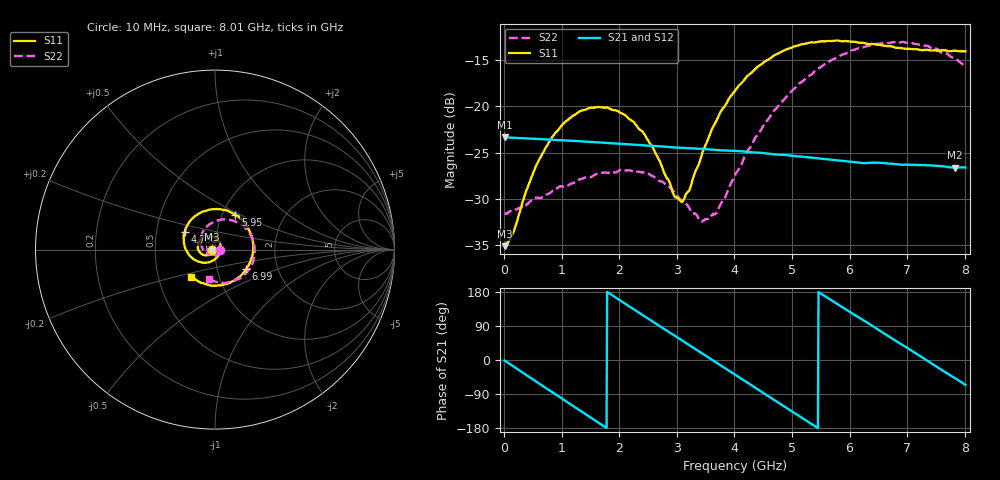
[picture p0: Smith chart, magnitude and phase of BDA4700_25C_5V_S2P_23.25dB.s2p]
!Agilent Technologies,E5071B,MY42404982,A.09.10
!Date: Mon Oct 20 13:38:07 2025
!Data & Calibration Information:
!Freq	S11:SOLT2(ON)	S21:SOLT2(ON)	S12:SOLT2(ON)	S22:SOLT2(ON)
# Hz S RI R 50
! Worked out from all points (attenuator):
!   801 points, 10 MHz to 8.01 GHz, reference 50 ohm
!   highest |S21| = -23.33 dB at 10 MHz (marker M1); lowest = -26.6 dB at 7.83 GHz (marker M2)
!   lowest |S11| = -35.2 dB at 10 MHz (marker M3), VSWR 1.04, Z = 48.3 - j0.102 ohm
!   |S11| at or under -10 dB: start of sweep to end of sweep
!   |S22| runs from -32.5 to -13.0 dB; largest |S21 - S12| = 0.00049
!   S11 on the Smith chart (normalised r, x): 10 MHz: 0.97, -0.00; 4.79 GHz: 0.70, +0.14; 5.95 GHz: 1.15, +0.47; 6.99 GHz: 1.38, -0.32; 8.01 GHz: 0.74, -0.23
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1e7  -0.0174 -0.00105  0.0682 -0.00146  0.0682 -0.00154  0.0262 -0.000834
1.6e8  -0.0183 -0.00974  0.0648 -0.0193  0.0648 -0.0193  0.0263 -0.0075
4.3e8  -0.0282 -0.0251  0.0482 -0.0466  0.0482 -0.0466  0.0196 -0.0227
7.3e8  -0.0508 -0.0322  0.0179 -0.0637  0.0179 -0.0638  0.00382 -0.033
1.35e9  -0.095 0.00575  -0.0469 -0.0445  -0.0469 -0.0445  -0.0364 -0.0177
2.09e9  -0.05 0.0751  -0.0541 0.0313  -0.0541 0.0314  -0.0289 0.0346
2.42e9  -0.0071 0.0717  -0.0282 0.0547  -0.0282 0.0547  -0.00428 0.0437
2.68e9  0.0198 0.0481  -0.00183 0.0608  -0.0019 0.0608  0.0136 0.0373
2.96e9  0.0311 0.00969  0.0259 0.054  0.026 0.0539  0.0261 0.022
3.1e9  0.0284 -0.0112  0.0379 0.0461  0.0378 0.0461  0.0284 0.0107
3.41e9  0.00121 -0.0515  0.0552 0.0204  0.0553 0.0204  0.0204 -0.0124
3.54e9  -0.017 -0.0638  0.0581 0.00763  0.0581 0.00757  0.0127 -0.0211
3.7e9  -0.0457 -0.0718  0.0575 -0.00815  0.0574 -0.00829  -0.00111 -0.0268
4.01e9  -0.1049 -0.0612  0.0449 -0.0357  0.0449 -0.0357  -0.033 -0.0263
4.79e9  -0.169 0.0988  -0.0233 -0.0495  -0.0231 -0.0497  -0.0793 0.0662
5.35e9  -0.0669 0.2117  -0.0519 -0.00913  -0.0519 -0.0093  -0.0155 0.1491
5.95e9  0.1139 0.1951  -0.0337 0.0376  -0.0338 0.0374  0.1207 0.1526
6.68e9  0.2118 -0.0137  0.0229 0.0433  0.0229 0.0434  0.2207 -0.00147
6.99e9  0.173 -0.1103  0.0406 0.0262  0.0407 0.0261  0.2041 -0.0851
7.43e9  0.0516 -0.1943  0.0471 -0.00802  0.0471 -0.0082  0.1177 -0.1691
7.83e9  -0.0811 -0.1835  0.0312 -0.0346  0.0311 -0.0348  0.0109 -0.1812
8.01e9  -0.1311 -0.15  0.0193 -0.0424  0.0195 -0.0425  -0.0324 -0.1613
